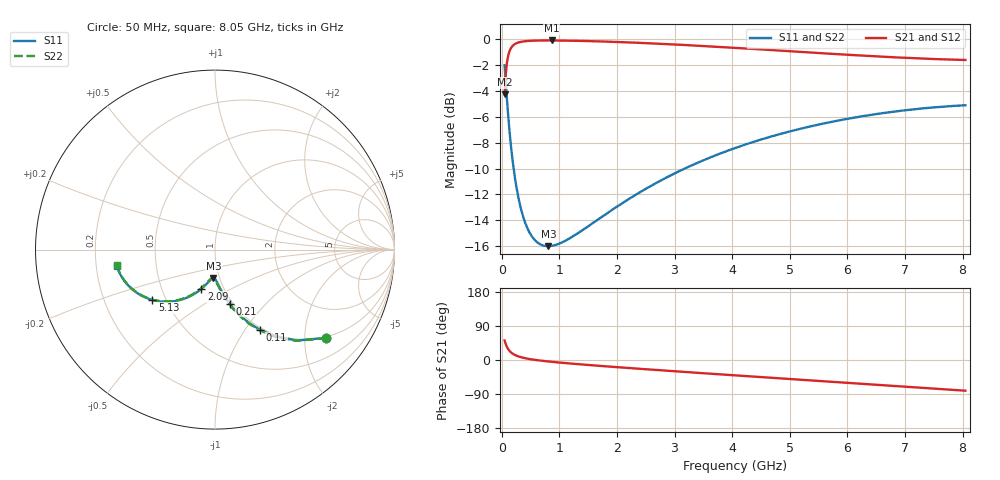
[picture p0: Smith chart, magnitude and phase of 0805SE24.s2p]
! AVX Thin Film Operation		Date: August 2001
! Description: Accu-P® Series, Thin Film, SMD, RF Capacitor
! Part Number: 08053J240FBW
! 50 MHz  -  8.05 GHz
! Serial Measurements
# mhz S db R 50
!	S11		S21		S12		S22
!	dB	Phase	dB	Phase	dB	Phase	dB	Phase
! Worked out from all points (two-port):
!   401 points, 50 MHz to 8.05 GHz, reference 50 ohm
!   highest |S21| = -0.11 dB at 870 MHz (marker M1); lowest = -4.3 dB at 50 MHz (marker M2)
!   |S21| within 3 dB of the highest: 64.91 MHz to end of sweep
!   lowest |S11| = -16.0 dB at 810 MHz (marker M3), VSWR 1.38, Z = 46.8 - j15.2 ohm
!   |S11| at or under -10 dB: 206.7 MHz to 3.177 GHz (2.97 GHz wide, 176 % of centre)
!   |S22| runs from -16.0 to -2.0 dB; largest |S21 - S12| = 9.6e-05
!   S11 on the Smith chart (normalised r, x): 50 MHz: 0.97, -2.55; 110 MHz: 0.97, -1.18; 210 MHz: 0.97, -0.65; 2.09 GHz: 0.78, -0.36; 5.13 GHz: 0.42, -0.30; 8.05 GHz: 0.29, -0.07
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50  -2.03 -38.4  -4.28 51.5  -4.28 51.5  -2.03 -38.5
70  -3.34 -48.1  -2.71 41.8  -2.71 41.8  -3.34 -48.3
110  -5.79 -60.7  -1.33 29.1  -1.33 29.1  -5.79 -61.0
130  -6.86 -64.8  -1.01 24.9  -1.01 24.9  -6.86 -65.3
150  -7.81 -68.1  -0.79 21.6  -0.79 21.6  -7.81 -68.6
170  -8.66 -70.8  -0.64 18.9  -0.64 18.9  -8.66 -71.3
210  -10.11 -74.8  -0.45 14.8  -0.45 14.8  -10.11 -75.5
250  -11.29 -77.8  -0.34 11.8  -0.34 11.8  -11.29 -78.5
310  -12.66 -81.0  -0.24 8.5  -0.24 8.5  -12.66 -81.9
370  -13.68 -83.4  -0.19 6.0  -0.19 6.0  -13.68 -84.4
450  -14.64 -85.9  -0.15 3.4  -0.15 3.4  -14.64 -87.0
610  -15.67 -89.6  -0.12 -0.3  -0.12 -0.3  -15.67 -90.9
810  -15.99 -93.1  -0.11 -3.9  -0.11 -3.9  -15.99 -94.4
870  -15.96 -94.0  -0.11 -4.8  -0.11 -4.8  -15.96 -95.4
1390  -14.79 -101.1  -0.15 -11.8  -0.15 -11.8  -14.79 -102.2
2090  -12.68 -109.3  -0.24 -19.9  -0.24 -19.9  -12.68 -110.2
2730  -11.00 -116.3  -0.36 -26.8  -0.36 -26.8  -11.00 -117.0
4050  -8.42 -130.2  -0.68 -40.5  -0.68 -40.5  -8.42 -130.7
5130  -6.99 -141.1  -0.98 -51.5  -0.98 -51.5  -6.99 -141.5
5390  -6.71 -143.8  -1.05 -54.1  -1.05 -54.1  -6.71 -144.1
6730  -5.65 -157.2  -1.40 -67.5  -1.40 -67.5  -5.65 -157.5
8050  -5.12 -170.8  -1.62 -81.0  -1.62 -81.0  -5.11 -171.0
